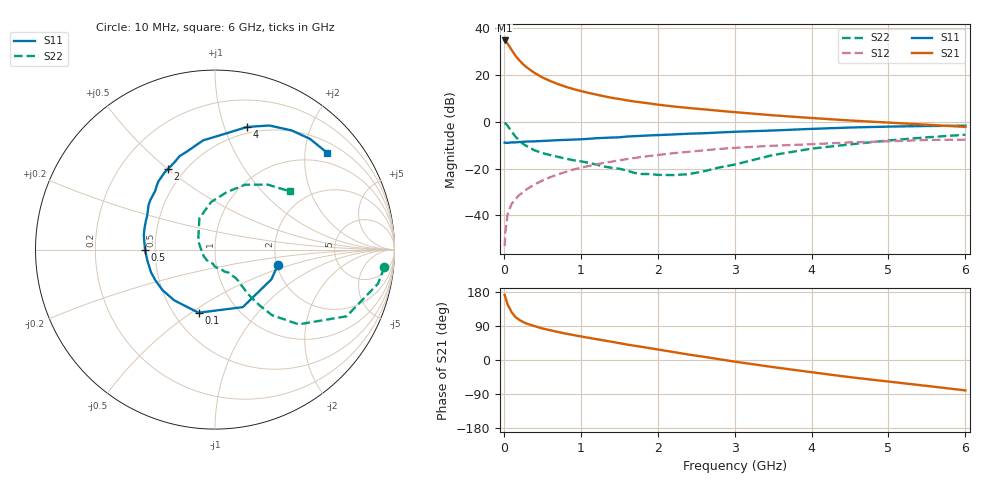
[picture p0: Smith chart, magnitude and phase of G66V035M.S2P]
! SIEMENS Small Signal Semiconductors
! BFG193
! Si NPN RF Bipolar Junction Transistor in SOT223
! VCE = 6 V  IC = 35 mA
! Common Emitter S-Parameters:  August  1996
# GHz  S  MA  R  50
!  f  S11  S21  S12  S22
! GHz  MAG  ANG  MAG  ANG  MAG  ANG  MAG  ANG
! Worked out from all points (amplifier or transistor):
!   36 points, 10 MHz to 6 GHz, reference 50 ohm
!   highest |S21| = 34.8 dB at 10 MHz (marker M1)
!   |S21| within 3 dB of that: start of sweep to 80.7 MHz
!   unconditionally stable (mu >= 1): 564.4 MHz to 2.407 GHz
!   at 250 MHz: K = 0.86, MSG = 27.3 dB, |S12| = -30.1 dB
!   at 1.4 GHz: K = 1.04, MAG = 12.4 dB, |S12| = -17.0 dB
!   at 6 GHz: K = 0.89, MSG = 2.7 dB, |S12| = -7.6 dB
!   S11 on the Smith chart (normalised r, x): 10 MHz: 2.02, -0.40; 100 MHz: 0.66, -0.53; 500 MHz: 0.44, -0.00; 2 GHz: 0.41, +0.50; 4 GHz: 0.44, +1.20; 6 GHz: 0.74, +2.49
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0.01  0.3606 -13.8  54.73 171.9  0.0022 86.9  0.9485 -5.9
0.02  0.3553 -27.8  53.38 165.3  0.0044 83.4  0.9279 -11.8
0.05  0.356 -64.2  46.51 146.1  0.0109 72.7  0.8216 -26.9
0.1  0.3635 -104.6  34.54 126.6  0.0175 65.4  0.6248 -41.8
0.15  0.3627 -128.7  26 113.5  0.0223 63.3  0.4838 -49.0
0.2  0.3695 -142.4  20.73 106.0  0.0271 64.6  0.3993 -51.3
0.25  0.374 -153.1  17.01 100.3  0.0314 64.9  0.3371 -52.8
0.3  0.3783 -160.6  14.45 95.9  0.0364 65.7  0.3002 -53.5
0.4  0.3821 -171.3  11.05 89.4  0.046 66.7  0.2458 -53.4
0.5  0.3896 -180.0  8.89 83.3  0.0553 66.1  0.2144 -53.3
0.6  0.3963 173.6  7.481 78.7  0.0652 65.3  0.1955 -54.0
0.8  0.4106 162.8  5.638 69.9  0.0847 62.8  0.1634 -57.5
1.1  0.4323 150.0  4.144 58.7  0.1136 58.1  0.1332 -66.7
1.6  0.4841 131.9  2.869 40.8  0.1597 47.8  0.0909 -92.0
2  0.5199 120.3  2.332 27.8  0.1953 39.2  0.0735 -132.4
2.2  0.5362 114.9  2.13 21.2  0.2127 34.7  0.0727 -149.8
2.8  0.5913 100.3  1.72 2.1  0.2628 21.0  0.1058 152.2
3.5  0.6517 84.2  1.377 -18.7  0.3081 4.0  0.1949 116.5
4  0.706 75.4  1.206 -32.2  0.3324 -5.8  0.2668 94.5
4.5  0.7546 66.4  1.066 -45.3  0.3632 -15.9  0.3292 78.0
5.5  0.8128 49.4  0.867 -68.4  0.4095 -39.2  0.4664 50.9
6  0.8251 40.9  0.778 -80.2  0.416 -52.6  0.5286 37.9
